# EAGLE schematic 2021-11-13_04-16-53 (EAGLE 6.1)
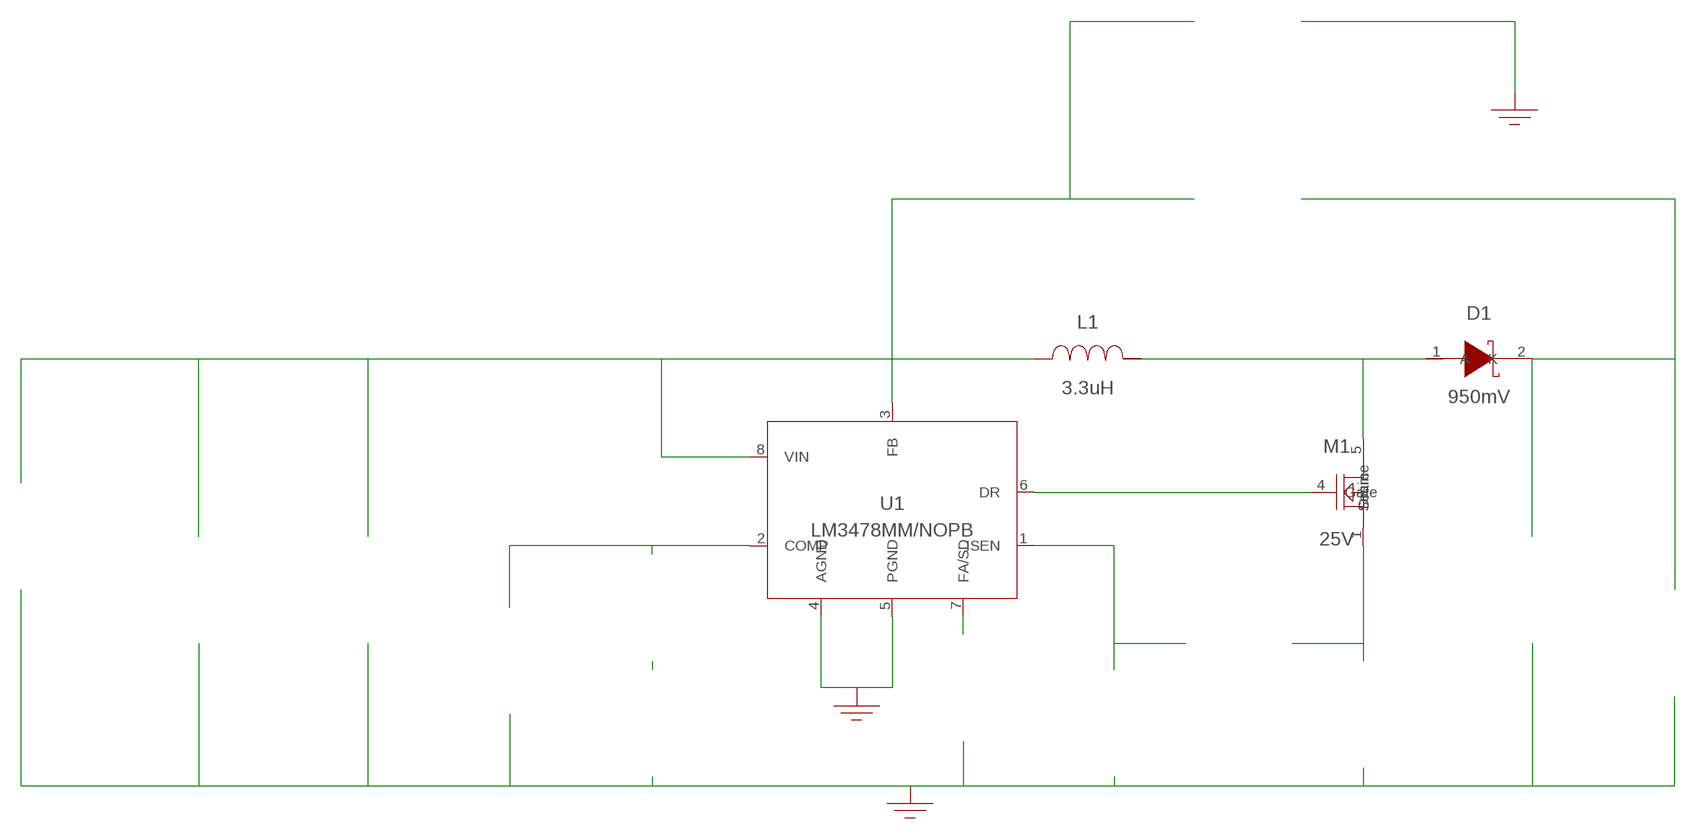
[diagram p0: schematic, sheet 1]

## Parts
CBYP  100nF  GRM155R70J104KA01DGRM155R70J104KA01D  [0402]  (not placed on a sheet)
CCOMP  47nF  C0805C473J3GACTUC0805C473J3GACTU  [0805]  (not placed on a sheet)
CCOMP2  2.7nF  C2012C0G1H272J060AAC2012C0G1H272J060AA  [0805]  (not placed on a sheet)
CFILT  10pF  CL21C100JBANNNCCL21C100JBANNNC  [0805]  (not placed on a sheet)
CIN  10uF  C0805C106K8PACTUC0805C106K8PACTU  [0805]  (not placed on a sheet)
COUT  56uF  CUSTOM1CUSTOM1  [GEN_Cap]  (not placed on a sheet)
D1  950mV  SBRD10200TRSBRD10200TR  [DPAK]
GND  WB_GND  WB_GNDWB_GND  [WB_GND]
GND2  WB_GND  WB_GNDWB_GND  [WB_GND]
GND_17  WB_GND  WB_GNDWB_GND  [WB_GND]
IOUT  WB_CURRENT_LOAD  WB_CURRENT_LOADWB_CURRENT_LOAD  [WB_CURRENT_LOAD]  (not placed on a sheet)
L1  3.3uH  SRP1270-3R3MSRP1270-3R3M  [SRP1270]
M1  25V  CSD16327Q3CSD16327Q3  [DQG0008A]
RCOMP  2.2k  RC0603FR-072K2LRC0603FR-072K2L  [0603]  (not placed on a sheet)
RFADJ  27k  RC0603FR-0727KLRC0603FR-0727KL  [0603]  (not placed on a sheet)
RFB1  101  RT0805BRD07101RLRT0805BRD07101RL  [0805]  (not placed on a sheet)
RFB2  1.5k  CRCW04021K50FKEDCRCW04021K50FKED  [0402]  (not placed on a sheet)
RFILT  100  CRCW0402100RFKEDCRCW0402100RFKED  [0402]  (not placed on a sheet)
RSENSE  10m  WSLP1206R0100FEAWSLP1206R0100FEA  [1206]  (not placed on a sheet)
U1  LM3478MM/NOPB  LM3478MM/NOPBLM3478MM/NOPB  [MUA08A]
VIN  WB_BATTERY  WB_BATTERYWB_BATTERY  [WB_BATTERY]  (not placed on a sheet)
Unconnected: CBYP.1 CBYP.2 CCOMP2.1 CCOMP2.2 CCOMP.1 CCOMP.2 CFILT.1 CFILT.2 CIN.1 CIN.2 COUT.1 COUT.2 D1.1(A) D1.2(K) D1.3(A) GND2.1 GND.1 GND_17.1 IOUT.1(+) IOUT.2(-) L1.1 L1.2 M1.1(Source) M1.2(Source) M1.3(Source) M1.4(Gate) M1.5(Drain) M1.6(Drain) M1.7(Drain) M1.8(Drain) M1.9(Drain) RCOMP.1 RCOMP.2 RFADJ.1 RFADJ.2 RFB1.1 RFB1.2 RFB2.1 RFB2.2 RFILT.1 RFILT.2 RSENSE.1 RSENSE.2 U1.1(ISEN) U1.2(COMP) U1.3(FB) U1.4(AGND) U1.5(PGND) U1.6(DR) U1.7(FA/SD) U1.8(VIN) VIN.1(+) VIN.2(-)

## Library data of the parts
CBYP = AcceleratedDesigns_Lib:GRM155R70J104KA01D; Manufacturer_Part_Number: GRM155R70J104KA01D; Vendor: MuRata
CCOMP = AcceleratedDesigns_Lib:C0805C473J3GACTU; Manufacturer_Part_Number: C0805C473J3GACTU; Vendor: Kemet
CCOMP2 = AcceleratedDesigns_Lib:C2012C0G1H272J060AA; Manufacturer_Part_Number: C2012C0G1H272J060AA; Vendor: TDK
CFILT = AcceleratedDesigns_Lib:CL21C100JBANNNC; Manufacturer_Part_Number: CL21C100JBANNNC; Vendor: Samsung Electro-Mechanics
CIN = AcceleratedDesigns_Lib:C0805C106K8PACTU; Manufacturer_Part_Number: C0805C106K8PACTU; Vendor: Kemet
COUT = AcceleratedDesigns_Lib:CUSTOM1; Manufacturer_Part_Number: GENERIC_CAPACITOR; Vendor: Unknown
D1 = AcceleratedDesigns_Lib:SBRD10200TR; Manufacturer_Part_Number: SBRD10200TR; Vendor: SMC Diode Solutions
GND GND2 GND_17 = AcceleratedDesigns_Lib:WB_GND; Manufacturer_Part_Number: WB_GND
IOUT = AcceleratedDesigns_Lib:WB_CURRENT_LOAD; Manufacturer_Part_Number: WB_CURRENT_LOAD
L1 = AcceleratedDesigns_Lib:SRP1270-3R3M; Manufacturer_Part_Number: SRP1270-3R3M; Vendor: Bourns
M1 = AcceleratedDesigns_Lib:CSD16327Q3; Manufacturer_Part_Number: CSD16327Q3; Vendor: Texas Instruments
RCOMP = AcceleratedDesigns_Lib:RC0603FR-072K2L; Manufacturer_Part_Number: RC0603FR-072K2L; Vendor: Yageo America
RFADJ = AcceleratedDesigns_Lib:RC0603FR-0727KL; Manufacturer_Part_Number: RC0603FR-0727KL; Vendor: Yageo America
RFB1 = AcceleratedDesigns_Lib:RT0805BRD07101RL; Manufacturer_Part_Number: RT0805BRD07101RL; Vendor: Yageo America
RFB2 = AcceleratedDesigns_Lib:CRCW04021K50FKED; Manufacturer_Part_Number: CRCW04021K50FKED; Vendor: Vishay-Dale
RFILT = AcceleratedDesigns_Lib:CRCW0402100RFKED; Manufacturer_Part_Number: CRCW0402100RFKED; Vendor: Vishay-Dale
RSENSE = AcceleratedDesigns_Lib:WSLP1206R0100FEA; Manufacturer_Part_Number: WSLP1206R0100FEA; Vendor: Vishay-Dale
U1 = AcceleratedDesigns_Lib:LM3478MM/NOPB; Manufacturer_Part_Number: LM3478MM/NOPB; Vendor: Texas Instruments
VIN = AcceleratedDesigns_Lib:WB_BATTERY; Manufacturer_Part_Number: WB_BATTERY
